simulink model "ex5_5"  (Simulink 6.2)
settings: Solver=ode45  SolverMode=SingleTasking  StartTime=0.0  StopTime=1000  MaxStep=10  RelTol=1e-3  AbsTol=1e-6
libraries: simulink x1

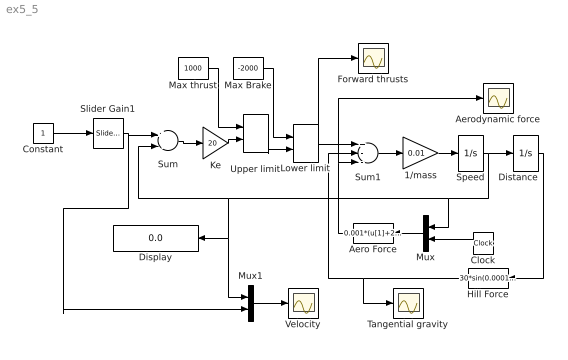
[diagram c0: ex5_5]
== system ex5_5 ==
  1/mass : Gain  Gain=0.01
  Aero Force : Fcn  Orientation=left  Expr=0.001*(u[1]+20*sin(0.01*u[2]))^2
  Aerodynamic force : Scope
  Clock : Clock
  Constant : Constant
  Display : Display
  Distance : Integrator
  Forward thrusts : Scope
  Hill Force : Fcn  Orientation=left  Expr=30*sin(0.0001*u[1])
  Ke : Gain  Gain=20
  Lower limit : MinMax  Function=max  Inputs=2
  Max Brake : Constant  Value=-2000
  Max thrust : Constant  Value=1000
  Mux : Mux  Orientation=left  Inputs=2
  Mux1 : Mux  Inputs=2
  Slider Gain1 : simulink/Math Operations/Slider Gain  low=0  gain=70  high=100
  Speed : Integrator
  Sum : Sum  Inputs=+-
  Sum1 : Sum  Inputs=+--
  Tangential gravity : Scope
  Upper limit : MinMax  Inputs=2
  Velocity : Scope
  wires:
  Speed/1 -> Distance/1, Mux/1, Display/1, Mux1/1, Sum/2
  Sum/1 -> Ke/1
  Mux/1 -> Aero Force/1
  Aero Force/1 -> Sum1/3, Aerodynamic force/1
  Hill Force/1 -> Sum1/2, Tangential gravity/1
  Distance/1 -> Hill Force/1
  Sum1/1 -> 1/mass/1
  1/mass/1 -> Speed/1
  Ke/1 -> Upper limit/2
  Upper limit/1 -> Lower limit/2
  Max thrust/1 -> Upper limit/1
  Max Brake/1 -> Lower limit/1
  Lower limit/1 -> Sum1/1, Forward thrusts/1
  Clock/1 -> Mux/2
  Constant/1 -> Slider Gain1/1
  Slider Gain1/1 -> Sum/1, Mux1/2
  Mux1/1 -> Velocity/1
